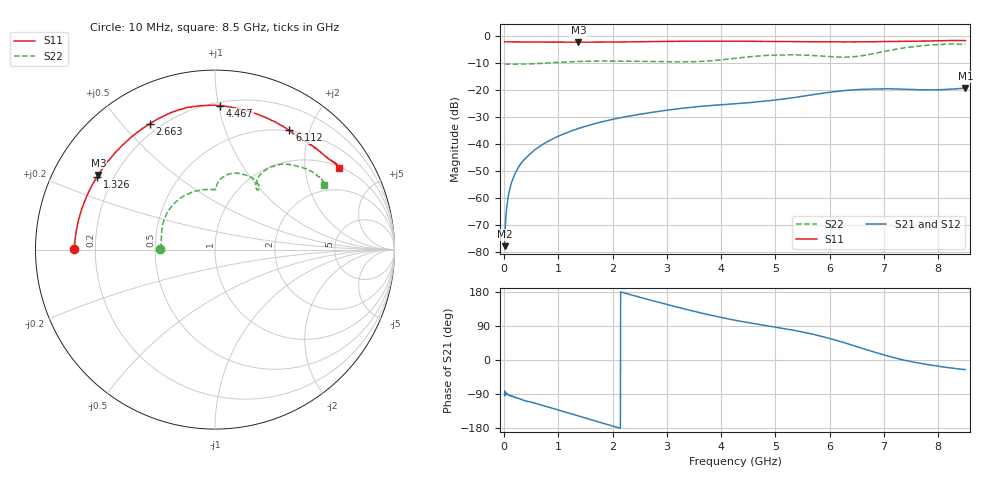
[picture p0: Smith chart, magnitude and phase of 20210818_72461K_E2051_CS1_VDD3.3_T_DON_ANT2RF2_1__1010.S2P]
!Agilent Technologies,E5071C,MY46417908,A.11.23
!Date: Wed Aug 18 14:26:44 2021
!Data & Calibration Information:
!Freq	S11:SOLT2(ON)	S21:SOLT2(ON)	S12:SOLT2(ON)	S22:SOLT2(ON)
!PortZ  Port1:50+j0  Port2:50+j0
!Above PortZ is port z conversion or system Z0 setting when saving the data.
!When reading, reference impedance value at option line is always used.
# Hz S dB R 50
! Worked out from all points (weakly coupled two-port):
!   1601 points, 10 MHz to 8.5 GHz, reference 50 ohm
!   highest |S21| = -19.27 dB at 8.5 GHz (marker M1); lowest = -77.8 dB at 10 MHz (marker M2)
!   lowest |S11| = -2.3 dB at 1.368 GHz (marker M3), VSWR 7.74, Z = 7 + j14.4 ohm
!   |S11| at or under -10 dB: nowhere
!   |S22| runs from -10.4 to -2.9 dB; largest |S21 - S12| = 0.00056
!   S11 on the Smith chart (normalised r, x): 10 MHz: 0.12, +0.00; 1.326 GHz: 0.14, +0.28; 2.663 GHz: 0.16, +0.60; 4.467 GHz: 0.23, +1.01; 6.112 GHz: 0.49, +1.69; 8.5 GHz: 1.06, +3.01
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1e7  -2.09 179.7  -77.76 -82.2  -78.86 -79.4  -10.34 179.6
6.30625e7  -2.13 178.5  -61.34 -90.5  -61.00 -90.9  -10.37 178.2
1.055125e8  -2.13 177.6  -56.55 -93.3  -56.58 -92.6  -10.38 177.0
1.798e8  -2.14 175.9  -51.92 -97.2  -51.99 -97.3  -10.40 174.8
2.965375e8  -2.16 173.2  -47.64 -102.6  -47.57 -102.5  -10.37 171.9
4.716438e8  -2.17 169.2  -43.77 -110.2  -43.74 -110.3  -10.29 167.6
6.998125e8  -2.19 163.7  -40.27 -119.4  -40.23 -119.5  -10.07 161.0
1.32595e9  -2.25 148.4  -34.51 -145.6  -34.52 -145.6  -9.42 140.3
1.3684e9  -2.26 147.4  -34.23 -147.4  -34.21 -147.4  -9.40 138.9
1.426769e9  -2.24 145.8  -33.81 -149.9  -33.83 -149.9  -9.36 136.7
2.663125e9  -2.05 117.3  -28.42 159.4  -28.42 159.4  -9.40 99.0
2.843538e9  -2.00 114.1  -27.89 152.5  -27.89 152.5  -9.44 95.7
4.255e9  -1.89 91.7  -25.04 105.0  -25.04 104.9  -8.24 86.2
4.46725e9  -1.92 88.0  -24.73 99.4  -24.74 99.5  -7.77 83.3
4.981956e9  -2.00 78.1  -23.68 87.1  -23.69 87.2  -7.03 72.2
5.671769e9  -2.09 64.9  -21.73 68.6  -21.74 68.8  -7.18 56.9
6.112188e9  -2.12 58.0  -20.53 52.3  -20.56 52.4  -7.71 54.4
6.610975e9  -2.13 51.4  -19.70 30.2  -19.72 30.1  -7.22 58.4
7.088538e9  -2.00 46.3  -19.51 9.9  -19.53 9.7  -5.33 56.9
7.449362e9  -1.94 42.6  -19.73 -2.6  -19.73 -2.6  -4.17 50.3
7.937538e9  -1.75 37.3  -19.87 -15.2  -19.86 -15.1  -3.18 38.7
8.5e9  -1.67 33.3  -19.27 -25.3  -19.27 -25.6  -3.02 30.7
